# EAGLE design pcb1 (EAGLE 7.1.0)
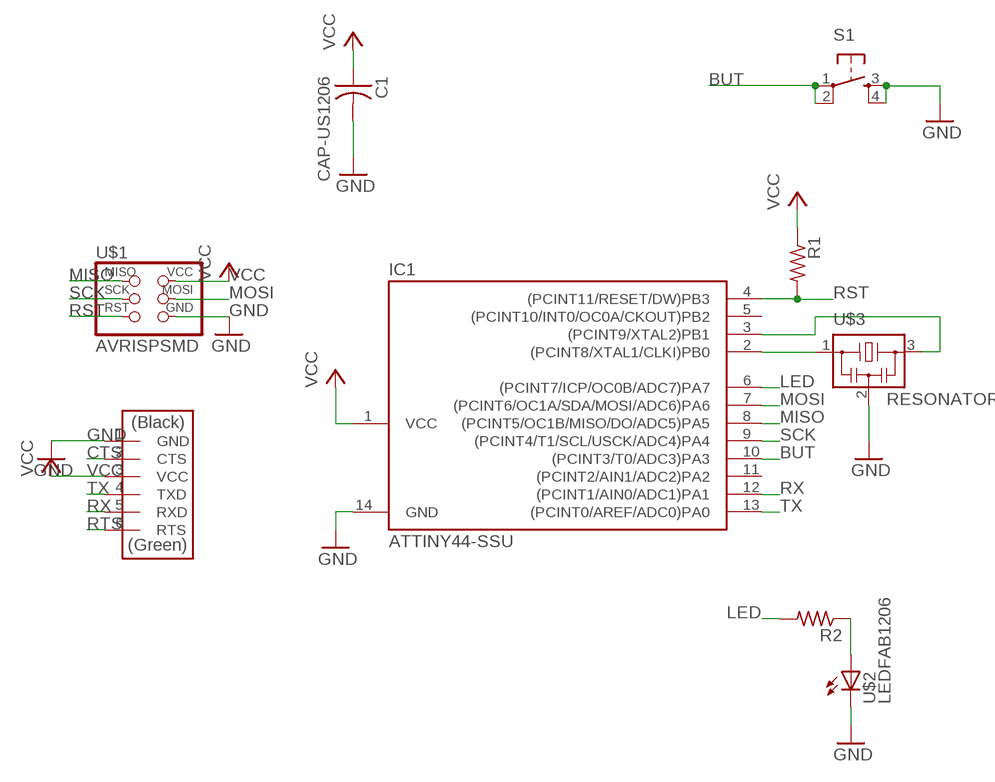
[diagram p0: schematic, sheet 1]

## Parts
C1  CAP-US1206  [C1206]
IC1  ATTINY44-SSU  [SOIC14]
R1  RES-US1206  [R1206]
R2  RES-US1206  [R1206]
RTS  FTDI-SMD-HEADER  [1X06SMD]
S1  6MM_SWITCH6MM_SWITCH  [6MM_SWITCH]
U$1  AVRISPSMD  [2X03SMD]
U$2  LEDFAB1206  [LED1206FAB]
U$3  RESONATOR  [EFOBM]

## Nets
BUT: IC1.10((PCINT3/T0/ADC3)PA3) S1.1(P) S1.2(P1)
CTS: RTS.2(CTS)
GND: C1.2 IC1.14(GND) RTS.1(GND) S1.3(S) S1.4(S1) U$1.6(GND) U$2.2(C) U$3.2
LED: IC1.6((PCINT7/ICP/OC0B/ADC7)PA7) R2.2
MISO: IC1.8((PCINT5/OC1B/MISO/DO/ADC5)PA5) U$1.1(MISO)
MOSI: IC1.7((PCINT6/OC1A/SDA/MOSI/ADC6)PA6) U$1.4(MOSI)
N$1: R2.1 U$2.1(A)
N$3: IC1.2((PCINT8/XTAL1/CLKI)PB0) U$3.1
N$4: IC1.3((PCINT9/XTAL2)PB1) U$3.3
RST: IC1.4((PCINT11/RESET/DW)PB3) R1.2 U$1.5(RST)
RTS: RTS.6(RTS)
RX: IC1.12((PCINT1/AIN0/ADC1)PA1) RTS.5(RXD)
SCK: IC1.9((PCINT4/T1/SCL/USCK/ADC4)PA4) U$1.3(SCK)
TX: IC1.13((PCINT0/AREF/ADC0)PA0) RTS.4(TXD)
VCC: C1.1 IC1.1(VCC) R1.1 RTS.3(VCC) U$1.2(VCC)
Unconnected: IC1.5((PCINT10/INT0/OC0A/CKOUT)PB2) IC1.11((PCINT2/AIN1/ADC2)PA2)

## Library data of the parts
C1 = fab:CAP-US
IC1 = fab:ATTINY44
R1 R2 = fab:RES-US: Resistor (US Symbol)
RTS = fab:FTDI-SMD-HEADER
S1 = fab:6MM_SWITCH: OMRON SWITCH
U$1 = fab:AVRISP
U$2 = fab:LED: LED
U$3 = fab:RESONATOR

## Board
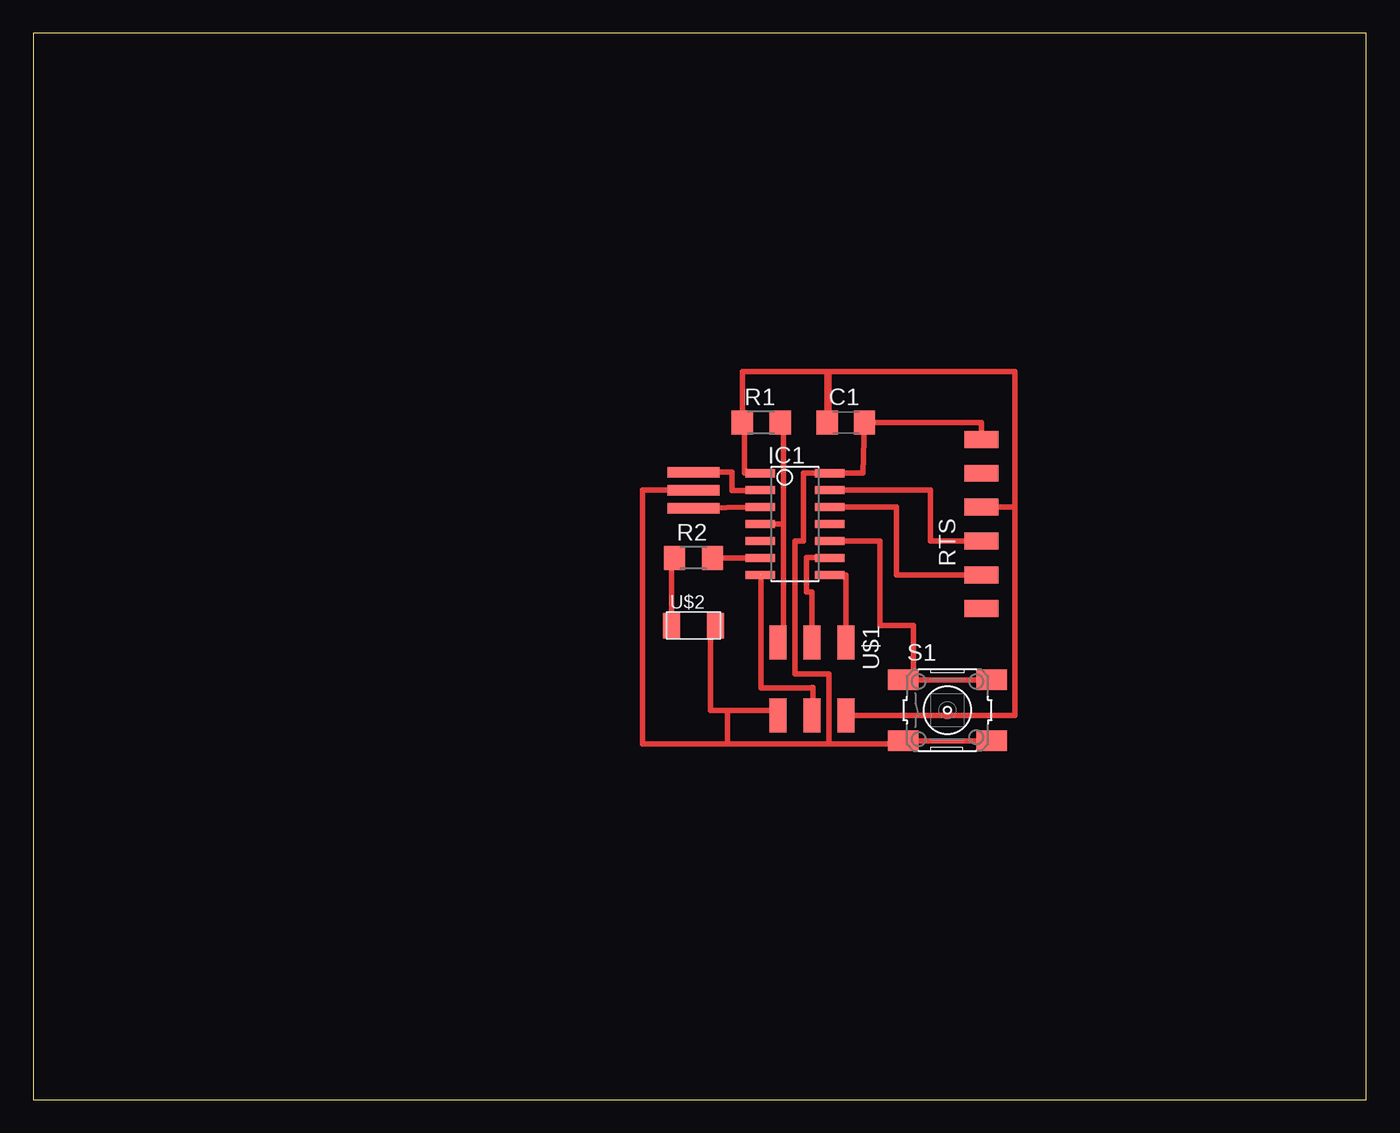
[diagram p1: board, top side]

Size 100 x 80 mm. Coordinates in mm from the lower left corner, seen from the top.
Outline: 0,0 100,0 100,80 0,80 0,0
Copper layers (1*16): Top 0.035mm / dielectric 1.5mm / Bottom 0.035mm
Design rules "default *": minimum track width 10mil, minimum drill 24mil, track to track 16mil, track to pad 16mil, pad to pad 8mil, via to via 8mil, smd to smd 8mil, copper to edge 40mil, drill to drill 8mil, minimum pad ring 10mil, minimum via ring 8mil, stop-mask expansion 4mil, vias tented up to drill 0mil, thermal gap 10mil

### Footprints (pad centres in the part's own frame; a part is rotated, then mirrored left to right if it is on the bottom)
C1206 = smd 1.6 x 1.8: 1 -1.4,0; 2 1.4,0
SOIC14 = smd 0.61 x 2.21: 1 -3.81,-2.603; 2 -2.54,-2.603; 3 -1.27,-2.603; 4 0,-2.603; 5 1.27,-2.603; 6 2.54,-2.603; 7 3.81,-2.603; 8 3.81,2.603; 9 2.54,2.603; 10 1.27,2.603; 11 0,2.603; 12 -1.27,2.603; 13 -2.54,2.603; 14 -3.81,2.603
R1206 = smd 1.6 x 1.803: 1 -1.422,0; 2 1.422,0
1X06SMD = smd 2.54 x 1.27: 1 0,6.35; 2 0,3.81; 3 0,1.27; 4 0,-1.27; 5 0,-3.81; 6 0,-6.35
6MM_SWITCH = smd 2.286 x 1.524: 1 -3.302,2.286; 2 3.302,2.286; 3 -3.302,-2.286; 4 3.302,-2.286
2X03SMD = smd 2.54 x 1.27: 1 -2.54,2.54; 2 2.92,2.54; 3 -2.54,0; 4 2.92,0; 5 -2.54,-2.54; 6 2.92,-2.54
LED1206FAB = smd 1.27 x 1.905: 1 -1.651,0; 2 1.651,0
EFOBM = smd 0.8 x 3.9: 1 -1.35,0; 2 0,0; 3 1.35,0

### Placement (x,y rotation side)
C1  60.96,50.8 0 top
IC1  57.15,43.18 270 top
R1  54.61,50.8 0 top
R2  49.53,40.64 0 top
RTS  71.12,43.18 0 top
S1  68.58,29.21 0 top
U$1  58.42,31.75 270 top
U$2  49.53,35.56 0 top
U$3  49.53,45.72 270 top

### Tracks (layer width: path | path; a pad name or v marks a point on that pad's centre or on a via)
BUT
  Top 0.406: S1.1 66.04,31.5 | 66.04,31.5 S1.2 | IC1.10 63.5,41.91 63.5,35.56 66.04,35.56 66.04,31.5
GND
  Top 0.406: S1.4 S1.3 65.28,26.67 59.7,26.67 | RTS.1 71.12,50.8 C1.2 62.23,46.99 IC1.14 57.77,46.99 57.77,41.91 57.15,41.91 57.15,31.92 59.7,31.92 59.7,26.67 | U$2.2 50.8,35.56 50.8,29.21 52.07,29.21 | 52.07,29.21 55.88,29.21 U$1.6 | U$3.2 45.72,45.72 45.72,26.67 52.07,26.67 | 52.07,26.67 59.7,26.67 | 52.07,29.21 52.07,26.67
LED
  Top 0.406: 50.8,40.64 R2.2 IC1.6
MISO
  Top 0.406: IC1.8 60.96,39.37 U$1.1
MOSI  (1 unrouted)
  Top 0.406: 54.61,39.37 54.61,31.75 54.58,31.75 54.58,30.87 58.42,30.87 58.42,30.93 58.48,30.93 58.48,29.75 58.42,29.75 U$1.4
N$1
  Top 0.406: R2.1 47.88,40.64 U$2.1
N$3
  Top 0.406: U$3.1 52.4,47.07 52.4,45.69 54.55,45.69 IC1.2
N$4
  Top 0.406: U$3.3 IC1.3
RST
  Top 0.406: 55.88,50.8 R1.2 56.27,50.8 | 56.52,50.8 56.27,50.8 | 56.27,50.8 56.27,43.19 | 55.88,43.19 54.61,43.19 54.61,43.18 | IC1.4 55.88,43.18 55.88,43.19 | 55.88,43.19 56.27,43.19 | 56.27,43.19 56.27,33.91 55.88,33.91 U$1.5
RX
  Top 0.406: RTS.5 64.77,39.37 64.77,44.45 IC1.12
SCK
  Top 0.406: U$1.3 58.42,38.1 58.02,38.1 58.02,38.11 58.01,38.11 58.01,40.66 59.75,40.66 IC1.9
TX
  Top 0.406: IC1.13 67.31,45.72 67.31,41.91 RTS.4
VCC
  Top 0.406: RTS.3 73.66,44.45 | 73.66,44.45 73.66,54.61 59.69,54.61 | 59.69,54.61 59.56,54.61 | 59.56,54.61 C1.1 59.69,50.8 59.69,54.61 | 59.56,54.61 53.19,54.61 R1.1 53.34,50.8 53.34,46.99 IC1.1 | U$1.2 73.66,28.83 73.66,44.45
